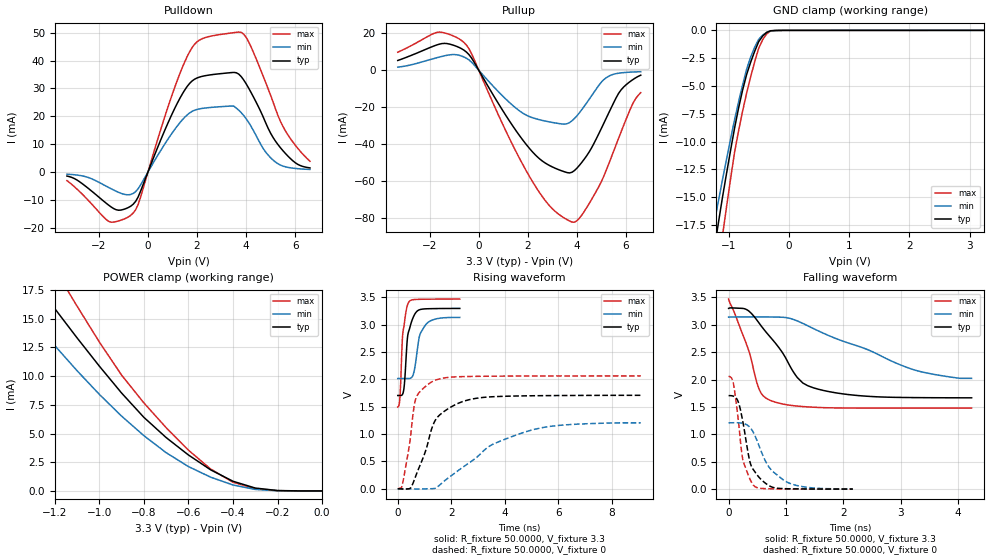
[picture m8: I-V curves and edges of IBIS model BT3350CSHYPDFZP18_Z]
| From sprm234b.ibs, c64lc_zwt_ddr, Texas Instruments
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[Model]   BT3350CSHYPDFZP18_Z
Model_type   I/O
Polarity   Non-Inverting
Enable   Active-Low
Vinl =  0.8V
Vinh =  2V
Cref =  15.0000pF
Rref =  100.0000M
Vref =  0V
Vmeas =  1.65
C_comp   1.700009p   1.65486p   1.747447p
[Model Spec]
Vinl   0.8V   0.8V   0.8V
Vinh   2V   2V   2V
[Temperature Range]   25   125   -40
[Voltage Range]   3.3   3.14   3.47
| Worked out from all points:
|   slope of the pulldown table from 0 to 0.495 V, typ, clamps not added: 45.1 ohm
|   slope of the pullup table from 0 to 0.495 V, typ, clamps not added: 43.8 ohm
|   GND clamp passes 1 mA (typ) near -0.50 V on its own axis
|   POWER clamp passes 1 mA (typ) near -0.42 V on its own axis
|   rising waveform, R_fixture 50.0000, V_fixture 3.3: 20-80 % time 204ps typ, 282ps min, 155ps max; typ from 1.71 V to 3.3 V
|   rising waveform, R_fixture 50.0000, V_fixture 0: 20-80 % time 851ps typ, 2.32ns min, 381ps max; typ from 0 V to 1.71 V
|   falling waveform, R_fixture 50.0000, V_fixture 3.3: 20-80 % time 668ps typ, 1.54ns min, 358ps max; typ from 3.3 V to 1.67 V
|   falling waveform, R_fixture 50.0000, V_fixture 0: 20-80 % time 218ps typ, 399ps min, 164ps max; typ from 1.71 V to 0.002 V
[POWER_clamp]
|   voltage   I(typ)   I(min)   I(max)
-3.3V     82.75mA    62.18mA    100.4mA
-1.4V     21.36mA    17.26mA    25.93mA
-1.367V   20.42mA    16.48mA    24.82mA
-1.233V   16.77mA    13.42mA    20.42mA
-1.133V   14.19mA    11.21mA    17.18mA
-900mV    8.53mA     6.519mA    10.09mA
-800mV    6.412mA    4.817mA    7.671mA
-600mV    3.133mA    2.123mA    3.553mA
-500mV    1.834mA    1.196mA    1.908mA
-400mV    842.6uA    517.5uA    755.5uA
-300mV    250.9uA    130.9uA    193.4uA
0V        112.1nA    206nA      236nA
[Pulldown]
|   voltage   I(typ)   I(min)   I(max)
-3.3V     -1.415mA   -746uA     -3.052mA
-1.6V     -11.86mA   -5.526mA   -17.66mA
-700mV    -12.23mA   -8.018mA   -15.5mA
-400mV    -8.953mA   -5.978mA   -11.65mA
900mV     19.24mA    12.9mA     25.53mA
1.7V      31.81mA    21.22mA    43.17mA
2.2V      34.3mA     22.8mA     47.78mA
3.7V      35.12mA    22.19mA    50.19mA
4.1V      30.16mA    17.85mA    46.75mA
5.1V      12.38mA    4.293mA    25.08mA
5.7V      5.755mA    1.687mA    13.38mA
6.6V      1.491mA    937.8uA    3.885mA
[Pullup]
|   voltage   I(typ)   I(min)   I(max)
-3.3V     5.278mA    1.679mA    9.743mA
-1.7V     13.72mA    6.799mA    20.48mA
-600mV    10.83mA    7.151mA    14.99mA
1.3V      -28.42mA   -18.04mA   -38.22mA
2.2V      -44.3mA    -25.71mA   -60.41mA
3V        -52.29mA   -28.23mA   -74.9mA
3.8V      -55.14mA   -27.3mA    -82.1mA
4.3V      -48.01mA   -19.44mA   -76.31mA
5.2V      -25.74mA   -3.982mA   -53.85mA
5.8V      -10.57mA   -1.415mA   -33.25mA
6.3V      -4.872mA   -941uA     -17.38mA
6.6V      -2.663mA   -794.7uA   -12.11mA
[GND_clamp]
|   voltage   I(typ)   I(min)   I(max)
-3.3V     -102mA     -77.67mA   -122mA
-1.3V     -22.05mA   -19.15mA   -26.55mA
-1.233V   -19.61mA   -17.23mA   -23.83mA
-1.167V   -17.27mA   -15.32mA   -21.14mA
-1.1V     -15.01mA   -13.43mA   -18.46mA
-1.033V   -12.88mA   -11.59mA   -15.88mA
-900mV    -8.803mA   -8.047mA   -10.98mA
-700mV    -3.977mA   -3.505mA   -5.648mA
-500mV    -1.023mA   -811uA     -1.621mA
-366.7mV  -182.6uA   -178.2uA   -313.2uA
-166.7mV  -5.411uA   -6.474uA   -7.343uA
3.233V    80.32nA    2.438uA    206.4nA
[Ramp]
| variable   typ   min   max
dV/dt_f  0.9852963/0.6653197n  0.7326568/1.726342n   1.20122/0.3596145n
dV/dt_r   1.031401/0.855675n   0.7444694/2.44115n   1.243471/0.3796375n
R_load = 50
[Rising Waveform]
R_fixture = 50.0000
V_fixture = 3.3
V_fixture_min = 3.14
V_fixture_max = 3.47
|   time   V(typ)   V(min)   V(max)
0s        1.706V     2.016V     1.495V
80ps      1.706V     2.017V     1.664V
168ps     1.719V     2.017V     2.695V
224ps     1.81V      2.017V     2.95V
352ps     2.706V     2.016V     3.342V
400ps     2.865V     2.016V     3.404V
576ps     3.133V     2.085V     3.458V
808ps     3.273V     2.784V     3.464V
1.04ns    3.29V      2.997V     3.466V
2.32ns    3.298V     3.134V     3.469V
[Rising Waveform]
R_fixture = 50.0000
V_fixture = 0
V_fixture_min = 0
V_fixture_max = 0
|   time   V(typ)   V(min)   V(max)
0s        45.56uV    24.27uV    73.91uV
136ps     -2.368mV   31.7uV     17.02mV
200ps     -6.367mV   30.4uV     139.7mV
488ps     20.4mV     -1.313mV   994.3mV
664ps     221.9mV    -4.669mV   1.63V
1.36ns    1.212V     4.288mV    1.976V
2.552ns   1.614V     434.5mV    2.053V
3.504ns   1.682V     801.3mV    2.059V
4.72ns    1.699V     1.032V     2.061V
9.088ns   1.709V     1.206V     2.064V
[Falling Waveform]
R_fixture = 50.0000
V_fixture = 3.3
V_fixture_min = 3.14
V_fixture_max = 3.47
|   time   V(typ)   V(min)   V(max)
0s        3.3V       3.14V      3.47V
344ps     3.258V     3.145V     2.552V
528ps     3.037V     3.145V     1.835V
704ps     2.805V     3.143V     1.632V
920ps     2.523V     3.139V     1.561V
1.2ns     2.037V     3.071V     1.517V
1.48ns    1.85V      2.931V     1.496V
2.216ns   1.713V     2.626V     1.481V
3.248ns   1.672V     2.174V     1.48V
4.24ns    1.668V     2.023V     1.481V
[Falling Waveform]
R_fixture = 50.0000
V_fixture = 0
V_fixture_min = 0
V_fixture_max = 0
|   time   V(typ)   V(min)   V(max)
0s        1.707V     1.212V     2.062V
88ps      1.696V     1.213V     1.908V
176ps     1.572V     1.212V     1.2V
224ps     1.364V     1.206V     709.1mV
256ps     1.191V     1.2V       505.4mV
368ps     518.1mV    1.134V     197.6mV
456ps     321.8mV    985.3mV    50.24mV
704ps     65.69mV    405.8mV    8.402mV
1.016ns   8.892mV    131.4mV    3.689mV
2.168ns   2.342mV    6.416mV    865.4uV
